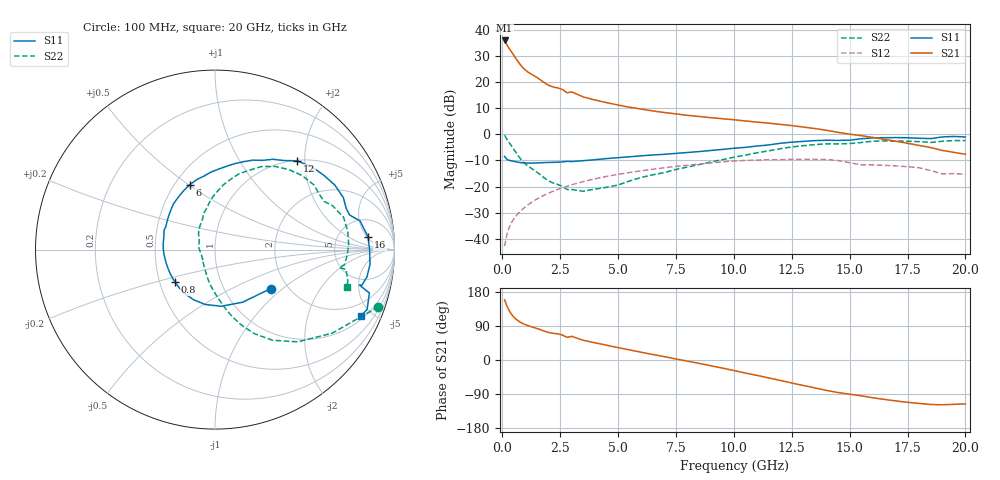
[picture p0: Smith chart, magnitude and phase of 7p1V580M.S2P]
! Infineon Technologies  Discrete & RF Semiconductors
! bfp620
! VCE =  1.5 V,  IC =  80 mA
! Common Emitter S-Parameters:  Sep 2002
# GHz  S  MA  R  50
!  f  S11  S21  S12  S22
! GHz  MAG  ANG  MAG  ANG  MAG  ANG  MAG  ANG
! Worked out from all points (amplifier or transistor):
!   59 points, 100 MHz to 20 GHz, reference 50 ohm
!   highest |S21| = 36.0 dB at 100 MHz (marker M1)
!   |S21| within 3 dB of that: start of sweep to 293.4 MHz
!   unconditionally stable (mu >= 1): 1.934 GHz to 2.333 GHz; 3.073 GHz to 10.01 GHz; 17.12 GHz to end of sweep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
!   at 1 GHz: K = 0.90, MSG = 26.2 dB, |S12| = -27.8 dB
!   at 5.5 GHz: K = 1.04, MAG = 11.3 dB, |S12| = -14.6 dB
!   at 20 GHz: K = 1.31, MAG = 0.5 dB, |S12| = -15.3 dB
!   S11 on the Smith chart (normalised r, x): 100 MHz: 1.64, -0.83; 800 MHz: 0.60, -0.24; 6 GHz: 0.59, +0.51; 12 GHz: 1.01, +1.84; 16 GHz: 10, +5; 20 GHz: 1.19, -4.31
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0.1  0.3788 -35.0  63.09 158.7  0.0072 80.5  0.9645 -19.3
0.2  0.3313 -62.2  51.84 142.6  0.0122 73.0  0.8021 -35.5
0.3  0.3175 -83.6  44.2 129.9  0.0166 70.1  0.6907 -48.1
0.4  0.3107 -99.9  38.03 120.3  0.0205 68.5  0.5983 -57.6
0.5  0.304 -113.0  32.65 113.0  0.0241 67.5  0.5162 -65.0
0.6  0.2974 -124.0  28.01 107.2  0.0275 66.9  0.4443 -70.8
0.7  0.2917 -133.2  24.15 102.7  0.0309 66.5  0.3839 -75.7
0.8  0.2875 -140.9  21.1 98.9  0.0342 66.1  0.3356 -79.8
0.9  0.2846 -147.3  18.77 95.8  0.0375 65.8  0.2983 -83.3
1.1  0.282 -157.1  15.76 90.9  0.0442 65.1  0.2486 -89.2
1.9  0.2889 177.4  9.249 74.4  0.0714 60.2  0.137 -111.9
2.8  0.3042 158.9  6.251 59.8  0.1018 52.4  0.0877 -142.5
3  0.3017 155.7  6.513 62.4  0.1082 50.6  0.0876 -141.0
3.5  0.3134 147.3  5.213 51.9  0.1248 45.7  0.0812 -162.0
6  0.3879 111.2  3.051 20.5  0.2006 20.7  0.1493 125.9
7  0.4149 98.3  2.623 8.9  0.2292 10.8  0.185 111.8
10.5  0.5641 61.8  1.809 -34.4  0.3166 -29.3  0.4002 77.6
12  0.6741 47.2  1.556 -53.8  0.3266 -47.1  0.531 60.7
13.5  0.7584 28.3  1.293 -73.6  0.3316 -65.7  0.6367 40.5
16  0.8562 4.7  0.875 -99.7  0.2609 -89.4  0.7387 14.1
17  0.8674 -5.5  0.739 -108.0  0.2483 -97.3  0.7452 2.3
20  0.8923 -24.4  0.416 -115.8  0.1718 -107.2  0.7627 -16.0
